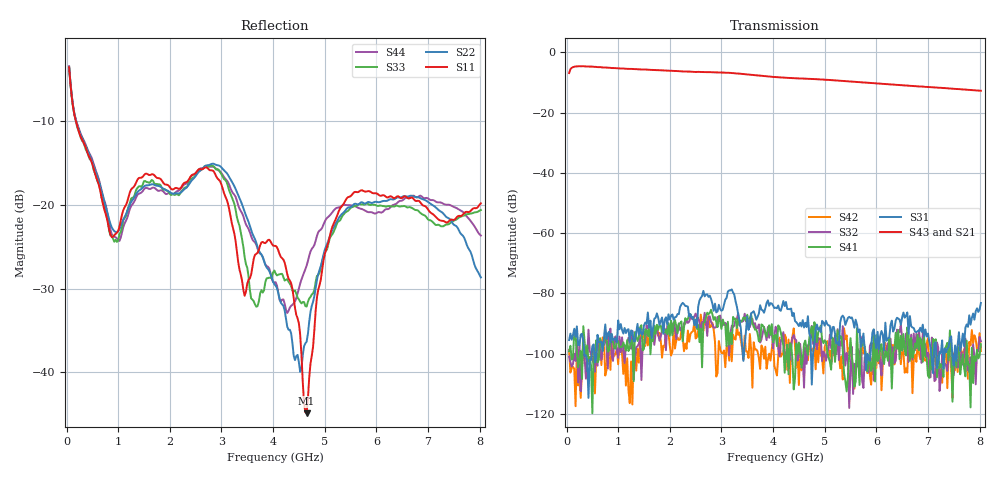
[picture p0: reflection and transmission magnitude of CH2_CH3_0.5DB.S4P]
!Agilent Technologies,E5071C,MY46316741,A.11.02
!Date: Thu May 28 14:38:43 2026
!Data & Calibration Information:
!1:CH2 INPUT 2:CH2 OUTPUT 3:CH3 INPUT 4:CH3 OUTPUT
!Freq	S11:SOLT4(ON)	S12:SOLT4(ON)	S13:SOLT4(ON)	S14:SOLT4(ON)
!	S21:SOLT4(ON)	S22:SOLT4(ON)	S23:SOLT4(ON)	S24:SOLT4(ON)
!	S31:SOLT4(ON)	S32:SOLT4(ON)	S33:SOLT4(ON)	S34:SOLT4(ON)
!	S41:SOLT4(ON)	S42:SOLT4(ON)	S43:SOLT4(ON)	S44:SOLT4(ON)
!PortZ  Port1:50+j0  Port2:50+j0  Port3:50+j0  Port4:50+j0
!Above PortZ is port z conversion or system Z0 setting when saving the data.
!When reading, reference impedance value at option line is always used.
# Hz S dB R 50
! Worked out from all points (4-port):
!   320 points, 50 MHz to 8.025 GHz, reference 50 ohm
!   strongest paths, dB at 50 MHz, 2.05 GHz, 4.05 GHz, 6.05 GHz, 8.025 GHz:
!     S43: -6.9, -6.2, -8.2, -10.4, -12.8
!     S21: -7.0, -6.3, -8.5, -10.6, -13.0
!     S31: -95.5, -87.0, -84.8, -98.5, -83.2
!     S41: -99.3, -94.0, -93.8, -101.9, -96.9
!     S32: -101.0, -90.8, -91.1, -99.0, -95.9
!     S42: -98.9, -99.4, -105.6, -103.3, -99.2
!   lowest |S11| = -44.9 dB at 4.65 GHz (marker M1), VSWR 1.01, Z = 50.5 + j0.259 ohm
!   |S11| at or under -10 dB: 182.7 MHz to end of sweep
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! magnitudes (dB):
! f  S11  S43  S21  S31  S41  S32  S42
! 50 MHz  -3.5  -6.9  -7.0  -95.5  -99.3  -101.0  -98.9
! 1 GHz  -23.1  -5.3  -5.5  -89.0  -95.9  -101.5  -103.6
! 2.85 GHz  -16.0  -6.7  -6.8  -85.8  -88.8  -91.4  -92.0
! 4.225 GHz  -26.9  -8.4  -8.7  -84.2  -106.4  -101.1  -93.7
! 4.65 GHz  -44.9  -8.8  -9.0  -91.2  -98.9  -103.4  -99.1
! 5.425 GHz  -19.2  -9.6  -9.8  -89.3  -112.5  -99.8  -94.0
! 8.025 GHz  -19.8  -12.8  -13.0  -83.2  -96.9  -95.9  -99.2
